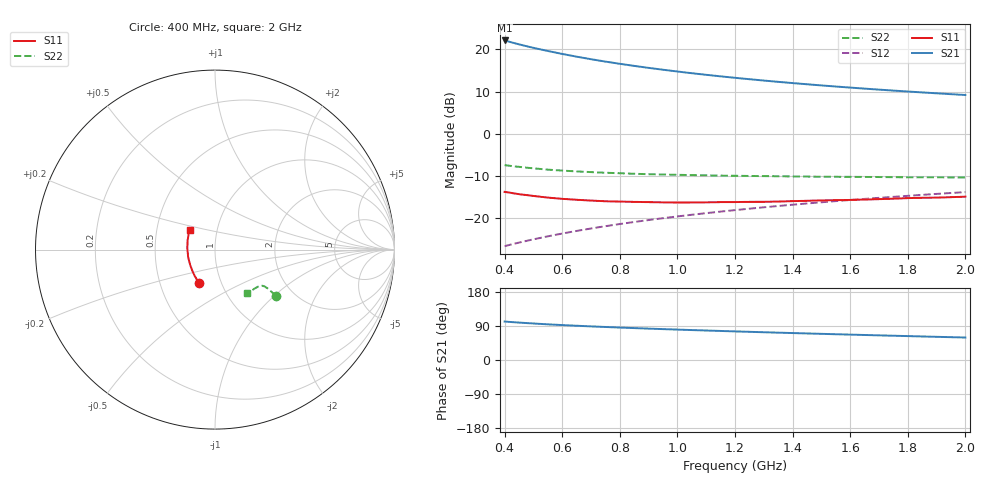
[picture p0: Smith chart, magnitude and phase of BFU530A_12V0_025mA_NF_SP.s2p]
! Filename:  P:\Prog\Test\Noise\ATS_data\Testdata_Net\06 Compressed Noise after Statistics\BFU530A_APG2013_33_A05_12p0V_025mA_NF_CM01_D.sf
! Date/Time: Tue 16/Apr/2013 15:11:00
! BFU530A_APG2013_33_A05_12p0V_1to25mA_NF_CM01_Bias8_R.sf
! Noise Parameter Data File
! BFU530A_APG2013_33_A05_12p0V_1to25mA_NF_CM01
! Date/time: Fri Apr 12 17:55:00 2013
! VAR V_out= 12.001000
! VAR I_out= 24.995000
! VAR V_in= 0.775500
! VAR I_in= 0.239250
! Device data file deembeded for feedlines and parallel
! Original file: \06 Compressed Noise after Statistics\BFU530A_APG2013_33_A05_12p0V_025mA_NF_CM01_R.sf
! Feed-files: PR017V01_150413_Feed1.s2p, PR017V01_150413_Feed2.s2p
! Parallel-file: PR017V01_150413_Par.s2p
# MHz S MA R 50
!  Freq-MHz  S11-mag  S11-arg  S21-mag  S21-arg  S12-mag  S12-arg  S22-mag  S22-arg
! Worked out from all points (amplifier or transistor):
!   37 points, 400 MHz to 2 GHz, reference 50 ohm
!   highest |S21| = 22.1 dB at 400 MHz (marker M1)
!   |S21| within 3 dB of that: start of sweep to 585.9 MHz
!   unconditionally stable (mu >= 1): 997.8 MHz to end of sweep
!   at 500 MHz: K = 0.93, MSG = 22.7 dB, |S12| = -25.0 dB
!   at 1.1 GHz: K = 1.00, MAG = 16.0 dB, |S12| = -18.8 dB
!   at 2 GHz: K = 1.00, MAG = 11.4 dB, |S12| = -13.8 dB
!   lowest NFmin = 1.21 dB at 480 MHz
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400  0.2044 -116.1  12.76 101.5  0.04643 72.2  0.4245 -37.1
420  0.1997 -119.0  12.21 100.3  0.04836 72.3  0.4157 -37.1
440  0.1943 -121.8  11.72 99.2  0.05025 72.5  0.4082 -36.9
480  0.1867 -126.7  10.83 97.3  0.05405 72.8  0.3946 -36.8
500  0.1829 -129.2  10.43 96.3  0.05597 72.9  0.389 -36.7
550  0.1749 -135.2  9.573 94.1  0.0607 73.2  0.3749 -36.5
600  0.169 -140.2  8.828 92.2  0.06555 73.4  0.3655 -36.4
650  0.1648 -145.2  8.195 90.4  0.07041 73.5  0.3575 -36.5
700  0.1613 -149.8  7.647 88.7  0.07525 73.5  0.3508 -36.5
750  0.1582 -154.3  7.164 87.1  0.08011 73.5  0.3446 -36.6
800  0.1569 -158.3  6.745 85.7  0.085 73.5  0.3401 -36.8
850  0.1556 -162.5  6.371 84.2  0.08986 73.4  0.3351 -37.1
900  0.1545 -166.3  6.036 82.8  0.09476 73.3  0.3312 -37.4
950  0.1536 -169.7  5.736 81.5  0.09965 73.2  0.3285 -37.9
1050  0.1531 -176.2  5.217 79.0  0.1095 72.9  0.3232 -38.7
1100  0.1536 -179.2  4.994 77.8  0.1144 72.7  0.3211 -39.2
1200  0.1548 175.0  4.602 75.5  0.1243 72.2  0.3173 -40.4
1350  0.157 167.2  4.122 72.2  0.139 71.3  0.3133 -42.4
1500  0.162 160.2  3.738 69.0  0.1539 70.4  0.3092 -44.6
1650  0.1657 154.1  3.425 66.0  0.1688 69.3  0.3072 -47.1
1750  0.1697 150.4  3.246 64.0  0.1785 68.6  0.3055 -48.8
2000  0.1793 142.2  2.878 59.3  0.2031 66.6  0.3032 -53.5
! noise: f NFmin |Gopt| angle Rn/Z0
400  1.252  0.2257  -167.2  0.1021
460  1.223  0.2578  -167.5  0.0891
600  1.315  0.2155  -159.7  0.1161
800  1.285  0.2605  -156.3  0.0986
1000  1.308  0.2781  -152.2  0.0969
1200  1.324  0.2787  -145.7  0.1099
1400  1.37  0.2929  -139.3  0.1135
1600  1.375  0.3093  -135.2  0.1185
1800  1.364  0.3294  -130.2  0.1245
2000  1.391  0.3358  -126.3  0.1363
